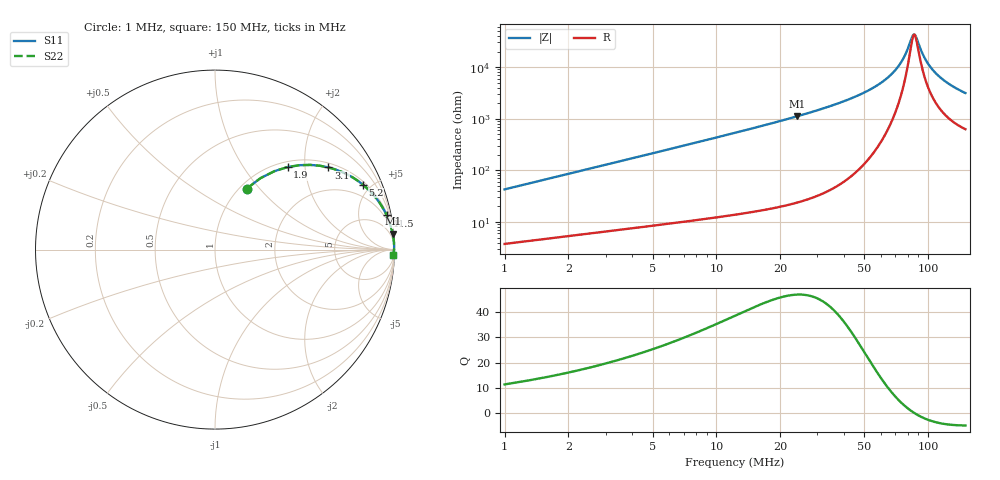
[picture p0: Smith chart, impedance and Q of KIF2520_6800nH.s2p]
!version-2
!date-12.2020
!Series
# MHz S RI R 50
!Freq ReS11 ImS11 ReS21 ImS21 ReS12 ImS12 ReS22 ImS22
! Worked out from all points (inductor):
!   498 points, 1 MHz to 150 MHz, reference 50 ohm
!   read as one part in series: L = 6.8 uH near 1.6 MHz
!   highest Q = 46.9 at 24.1 MHz (marker M1), where L = 7.38 uH
!   self-resonance near 85.9 MHz
!   S11 on the Smith chart (normalised r, x): 1 MHz: 1.08, +0.85; 1.9 MHz: 1.10, +1.62; 3.1 MHz: 1.13, +2.65; 5.2 MHz: 1.17, +4.46; 11.5 MHz: 1, +10; 150 MHz: 14, -62
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1  0.176 0.3393  0.824 -0.3393  0.824 -0.3393  0.176 0.3393
1.9  0.4044 0.4598  0.5956 -0.4598  0.5956 -0.4598  0.4044 0.4598
3.1  0.6318 0.4579  0.3682 -0.4579  0.3682 -0.4579  0.6318 0.4579
4  0.737 0.4187  0.263 -0.4187  0.263 -0.4187  0.737 0.4187
5.2  0.8234 0.3624  0.1766 -0.3624  0.1766 -0.3624  0.8234 0.3624
7.6  0.9074 0.2743  0.0926 -0.2743  0.0926 -0.2743  0.9074 0.2743
11.5  0.9569 0.1901  0.0431 -0.1901  0.0431 -0.1901  0.9569 0.1901
16.9  0.9797 0.13  0.0203 -0.13  0.0203 -0.13  0.9797 0.13
24.1  0.9902 0.0884  0.00979 -0.0884  0.00979 -0.0884  0.9902 0.0884
25.9  0.9916 0.0813  0.00841 -0.0813  0.00841 -0.0813  0.9916 0.0813
50.8  0.9978 0.0299  0.00219 -0.0299  0.00219 -0.0299  0.9978 0.0299
65.8  0.9982 0.0147  0.00182 -0.0147  0.00182 -0.0147  0.9982 0.0147
75.7  0.998 0.00698  0.00197 -0.00698  0.00197 -0.00698  0.998 0.00698
79.3  0.9979 0.00446  0.00207 -0.00446  0.00207 -0.00446  0.9979 0.00446
84.1  0.9978 0.00128  0.00225 -0.00128  0.00225 -0.00128  0.9978 0.00128
85.9  0.9977 0.000146  0.00232 -0.000146  0.00232 -0.000146  0.9977 0.000146
87.7  0.9976 -0.000969  0.0024 0.000969  0.0024 0.000969  0.9976 -0.000969
94.6  0.9973 -0.00504  0.00275 0.00504  0.00275 0.00504  0.9973 -0.00504
100.6  0.9969 -0.00835  0.0031 0.00835  0.0031 0.00835  0.9969 -0.00835
111.1  0.9962 -0.0137  0.0038 0.0137  0.0038 0.0137  0.9962 -0.0137
125.2  0.9951 -0.0204  0.00491 0.0204  0.00491 0.0204  0.9951 -0.0204
150  0.9927 -0.0307  0.00726 0.0307  0.00726 0.0307  0.9927 -0.0307
